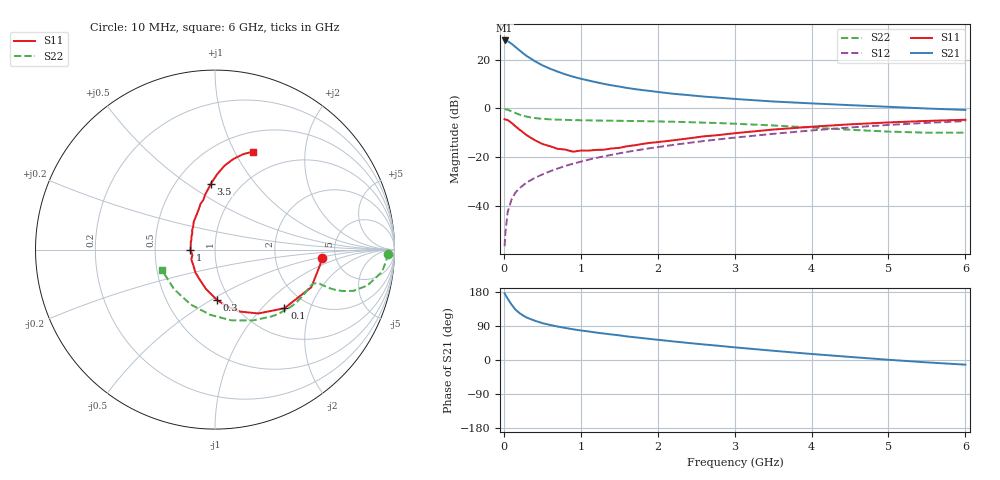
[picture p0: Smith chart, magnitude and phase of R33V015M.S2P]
! SIEMENS Small Signal Semiconductors
! BFR181
! Si NPN RF Bipolar Junction Transistor in SOT23
! VCE = 3 V  IC = 15 mA
! Common Emitter S-Parameters:  May  1996
# GHz  S  MA  R  50
!  f  S11  S21  S12  S22
! GHz  MAG  ANG  MAG  ANG  MAG  ANG  MAG  ANG
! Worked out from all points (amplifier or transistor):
!   36 points, 10 MHz to 6 GHz, reference 50 ohm
!   highest |S21| = 27.8 dB at 10 MHz (marker M1)
!   |S21| within 3 dB of that: start of sweep to 163.2 MHz
!   unconditionally stable (mu >= 1): 506.3 MHz to 2.633 GHz
!   at 250 MHz: K = 0.76, MSG = 27.1 dB, |S12| = -31.5 dB
!   at 1.4 GHz: K = 1.10, MAG = 12.4 dB, |S12| = -19.0 dB
!   at 6 GHz: K = 0.87, MSG = 2.3 dB, |S12| = -5.2 dB
!   S11 on the Smith chart (normalised r, x): 10 MHz: 3.88, -0.59; 100 MHz: 1.54, -1.35; 300 MHz: 0.87, -0.53; 1 GHz: 0.76, -0.00; 3.5 GHz: 0.73, +0.62; 6 GHz: 0.71, +1.19
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0.01  0.5984 -4.7  24.67 176.0  0.0015 88.0  0.9641 -1.3
0.02  0.5914 -8.5  24.4 172.2  0.0028 87.3  0.959 -3.0
0.05  0.5761 -21.3  23.75 161.7  0.0075 80.1  0.939 -7.6
0.1  0.5064 -40.2  21.13 146.3  0.0136 74.7  0.8717 -13.3
0.15  0.43 -55.9  18.17 133.3  0.0187 70.5  0.8046 -16.6
0.2  0.3712 -68.3  15.63 124.4  0.0229 69.6  0.747 -18.0
0.25  0.3217 -78.4  13.49 117.4  0.0265 67.7  0.706 -18.5
0.3  0.2809 -87.8  11.79 111.8  0.0305 69.3  0.6757 -18.6
0.4  0.2239 -103.3  9.332 103.9  0.0374 70.3  0.6348 -18.3
0.5  0.1865 -117.5  7.645 97.3  0.0442 71.7  0.6119 -18.1
0.6  0.168 -130.3  6.514 92.6  0.0513 72.0  0.5965 -18.3
0.7  0.1483 -145.0  5.661 88.2  0.0586 72.6  0.587 -18.7
0.8  0.1429 -157.9  4.983 84.5  0.0661 72.5  0.581 -19.1
1  0.1367 -179.1  4.052 78.0  0.0809 73.0  0.5713 -20.5
1.1  0.1362 173.0  3.727 75.3  0.0889 73.2  0.5679 -21.5
1.3  0.1423 157.2  3.179 69.9  0.1042 72.4  0.5609 -23.6
1.6  0.1673 139.5  2.628 62.2  0.128 71.4  0.5534 -27.2
2.2  0.2214 117.3  1.993 49.1  0.1784 67.9  0.5324 -36.0
3.5  0.3683 93.5  1.385 24.4  0.3008 56.7  0.4468 -62.1
4.5  0.471 83.5  1.165 8.1  0.4063 44.9  0.3646 -94.1
5.5  0.5534 73.7  0.994 -6.3  0.5046 31.0  0.3174 -136.0
6  0.5849 68.9  0.93 -12.3  0.5479 23.4  0.3165 -158.5
